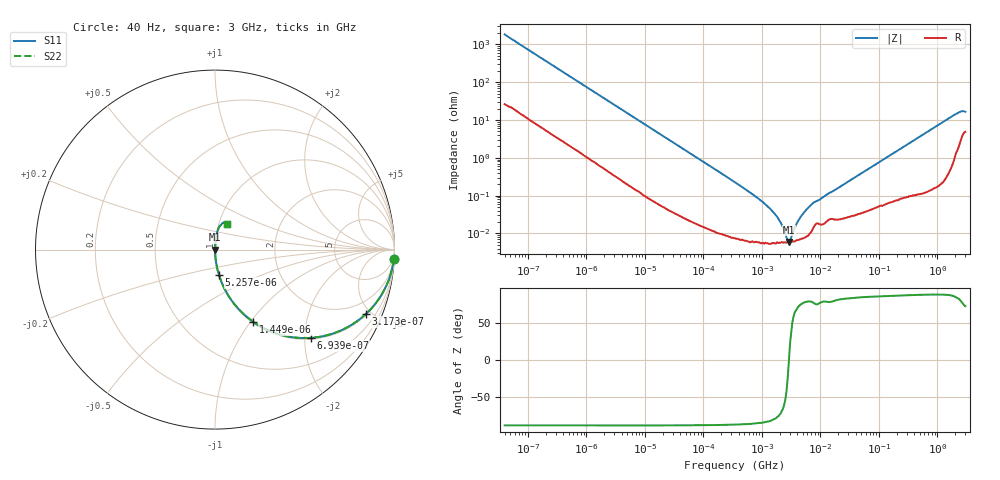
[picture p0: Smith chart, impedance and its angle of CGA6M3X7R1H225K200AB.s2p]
! S-parameter Generated by TDK Corporation
! Copyright(C) 2015 TDK Corporation.
! All Rights Reserved.
! TDK P/N: CGA6M3X7R1H225K200AB (Multilayer Ceramic Chip Capacitors)
! Property: C=2.2uF
! Size(LxWxT): 3.2x2.5x2mm, 0.126x0.098x0.079inches
! Model Type: s2p (Touchstone File Format Version 1.0)
! Frequency: DC=Yes Start=0.00004MHz Stop=3000MHz 396points Log-sweep
! Note: This model was converted from impedance.
! Model Generated on Jun. 23, 2015
! Hash(MD5):
! Port Assignments:
!  1 ---| |--- 2
! Applicable Conditions:
!  Temperature = 25 degC
!  DC Bias Voltage = 0 V
!  Small Signal Operation
! Terms and conditions regarding TDK Simulation Models
! (1)This simulation model is being provided solely for informational purposes. Please refer to the specifications of the products in terms of detailed characteristics of such products.
! (2)In no event shall TDK Corporation of any of its subsidiaries be liable for any loss or damage arising, directly or indirectly,
!  From any information contained in this simulation model, including, but not limited to loss or damages arising from any inaccuracies, omissions or errors in connection with such information.
! (3)Any and all copyrights on this simulation model are owned by TDK Corporation.
!  Duplication or redistribution of this simulation model without prior written permission from TDK Corporation is prohibited.
! (4)This simulation model is subject to any modification or change without any prior notice.
! (5)Neither TDK Corporation nor any of its subsidiaries shall make any warranty, express or implied,
!  Including but not limited to the correctness, implied warranties of merchantability and fitness for a particular purpose with respect to this simulation models.
! (6)The use of this simulation model shall be deemed to have consented to the terms and conditions hereof.
# MHz S MA R 50
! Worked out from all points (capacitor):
!   395 points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, 40 Hz to 3 GHz, reference 50 ohm
!   read as one part in series: C = 2.19 uF near 41.88 Hz
!   lowest |Z| = 5.97 mohm at 2.877 MHz (marker M1)
!   series resonance near 2.899 MHz, so ESL is about 1.4 nH
!   S11 on the Smith chart (normalised r, x): 40 Hz: 2, -36; 317.3 Hz: 1.07, -4.65; 693.9 Hz: 1.03, -2.14; 1.449 kHz: 1.01, -1.03; 5.257 kHz: 1.00, -0.29; 3 GHz: 1.10, +0.31
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4e-05  0.9977 -3.1  0.05478 86.0  0.05478 86.0  0.9977 -3.1
0.0001451139  0.9782 -11.2  0.1937 78.0  0.1937 78.0  0.9782 -11.2
0.0003173189  0.9139 -23.1  0.3928 66.0  0.3928 66.0  0.9139 -23.1
0.0006938775  0.7259 -42.6  0.6774 46.5  0.6774 46.5  0.7259 -42.6
0.000834128  0.6614 -47.8  0.7406 41.4  0.7406 41.4  0.6614 -47.8
0.001449046  0.4568 -62.0  0.8833 27.2  0.8833 27.2  0.4568 -62.0
0.002517282  0.2861 -72.6  0.9543 16.6  0.9543 16.6  0.2861 -72.6
0.005256919  0.1433 -81.0  0.9878 8.2  0.9878 8.2  0.1433 -81.0
0.01739424  0.04438 -86.7  0.9984 2.5  0.9984 2.5  0.04438 -86.7
0.3464102  0.002261 -88.0  0.9999 0.1  0.9999 0.1  0.002261 -88.0
1.256723  0.0005192 -83.9  0.9999 0.0  0.9999 0.0  0.0005192 -83.9
1.816098  0.000277 -77.8  0.9999 0.0  0.9999 0.0  0.000277 -77.8
2.183178  0.0001694 -69.6  0.9999 0.0  0.9999 0.0  0.0001694 -69.6
2.506407  9.991e-05 -54.4  0.9999 0.0  0.9999 0.0  9.991e-05 -54.4
2.877491  5.972e-05 -4.0  0.9999 0.0  0.9999 0.0  5.972e-05 -4.0
3.303516  9.583e-05 50.4  0.9999 -0.0  0.9999 -0.0  9.583e-05 50.4
4.5592  0.0002718 75.0  0.9999 -0.0  0.9999 -0.0  0.0002718 75.0
7.22376  0.000607 78.4  0.9999 -0.0  0.9999 -0.0  0.000607 78.4
150.6385  0.01133 86.1  0.9993 -0.6  0.9993 -0.6  0.01133 86.1
1982.595  0.1366 77.8  0.9804 -7.8  0.9804 -7.8  0.1366 77.8
2495.579  0.1605 70.9  0.9596 -9.1  0.9596 -9.1  0.1605 70.9
3000  0.1553 64.2  0.9429 -8.5  0.9429 -8.5  0.1553 64.2
